| IBIS file was generated by Viper version: 2024.10.21
[IBIS Ver]   4.2
[Comment Char]   |_char
[File Name]   mcxl20_100lqfp_14x14_l25x_tfme.ibs
[File Rev]   1.0
[Date]   Thu Oct 24 12:27:42 2024
[Source]   NXP Viper 2024.10.21
[Notes]
[Disclaimer] IMPORTANT NOTICE
  This information is provided on an AS IS basis and without warranty.
  IN NO EVENT SHALL NXP BE LIABLE FOR INCIDENTAL OR CONSEQUENTIAL
  DAMAGES ARISING FROM USE OF THIS INFORMATION. THIS DISCLAIMER OF
  WARRANTY EXTENDS TO THE USER OF THE INFORMATION, AND TO THEIR CUSTOMERS
  OR USERS OF PRODUCTS  AND IS IN LIEU OF ALL WARRANTIES WHETHER EXPRESS,
  IMPLIED, OR STATUTORY, INCLUDING IMPLIED WARRANTIES OF MERCHANTABILITY
  OR FITNESS FOR PARTICULAR PURPOSE.
  NXP does not represent or warrant that the information furnished
  hereunder is free of infringement of any third party patents,
  copyrights, trade secrets, or other intellectual property rights.
  NXP does not represent or warrant that the information is free of
  defect, or that it meets any particular standard, requirements or need
  of the user of the infomation or their customers.
  NXP reserves the right to change the information in this file
  without notice.
   http://www.nxp.com
[Copyright]   (C) Copyright NXP 2004 - 2024, All Rights Reserved.
|   MCXL20_100LQFP_14x14_L25x_TFME
[Component]   MCXL20_100LQFP_14x14_L25x_TFME
[Manufacturer]   NXP
[Package]
| variable   typ   min   max
R_pkg   0.30564   0.12887   0.35737
L_pkg   5.061e-09   3.022e-09   6.217e-09
C_pkg   1.277e-12   9.885e-13   1.603e-12
[Pin] signal_name   model_name   R_pin   L_pin   C_pin
1   P1_15   a_ip_io_3v_3p3v   0.34361   5.739e-09 1.392e-12
2   P1_16   a_ip_io_3v_3p3v   0.33129   5.397e-09 1.564e-12
3   P1_17   a_ip_io_3v_3p3v   0.33122   5.046e-09 1.446e-12
4   VDD   POWER   NA   NA   NA
5   P1_18   a_ip_io_3v_3p3v   0.33259   4.954e-09 1.335e-12
6   P1_19   a_ip_io_3v_3p3v   0.32237   5.168e-09 1.289e-12
7   P1_20   a_ip_io_3v_3p3v   0.30216   5.026e-09 1.237e-12
8   P1_21   a_ip_io_3v_3p3v   0.29683   4.978e-09 1.206e-12
9   P1_22   a_ip_io_3v_3p3v   0.29435   4.952e-09 1.177e-12
10   P2_0   a_ip_io_3v_3p3v   0.29406   4.947e-09 1.149e-12
11   P2_1   a_ip_io_3v_3p3v   0.29668   4.979e-09 1.095e-12
12   P2_2   a_ip_io_3v_3p3v   0.30138   4.867e-09 1.083e-12
13   P2_3   a_ip_io_3v_3p3v   0.30845   4.904e-09 1.063e-12
14   P2_4   a_ip_io_3v_3p3v   0.30483   4.804e-09 9.885e-13
15   P2_5   a_ip_io_3v_3p3v   0.30153   4.504e-09 1.003e-12
16   VDD   POWER   NA   NA   NA
17   VSS   GND   NA   NA   NA
18   VDD_CORE_FIXED   POWER   NA   NA   NA
19   P2_6   a_ip_io_3v_3p3v   0.31199   4.646e-09 1.139e-12
20   P2_7   a_ip_io_3v_3p3v   0.31342   4.987e-09 1.226e-12
21   P2_10   a_ip_io_3v_3p3v   0.30413   5.068e-09 1.266e-12
22   P2_11   a_ip_io_3v_3p3v   0.31487   5.260e-09 1.245e-12
23   P2_12   a_ip_io_3v_3p3v   0.31693   5.315e-09 1.349e-12
24   P2_13   a_ip_io_3v_3p3v   0.31822   5.354e-09 1.506e-12
25   P2_14   a_ip_io_3v_3p3v   0.33148   5.617e-09 1.387e-12
26   P2_15   a_ip_io_3v_3p3v   0.33786   5.719e-09 1.380e-12
27   P2_16   a_ip_io_3v_3p3v   0.31339   5.264e-09 1.544e-12
28   P2_17   a_ip_io_3v_3p3v   0.3118   5.209e-09 1.436e-12
29   P2_18   a_ip_io_3v_3p3v   0.30788   5.060e-09 1.333e-12
30   P2_19   a_ip_io_3v_3p3v   0.31046   4.771e-09 1.313e-12
31   VDD   POWER   NA   NA   NA
32   VDD_CORE_FIXED   POWER   NA   NA   NA
33   P2_20   NC   0.29722   4.575e-09 1.197e-12
34   P2_21   a_ip_io_3v_3p3v   0.29247   4.706e-09 1.175e-12
35   P2_22   a_ip_io_3v_3p3v   0.29166   4.730e-09 1.148e-12
36   P2_23   a_ip_io_3v_3p3v   0.29368   4.774e-09 1.094e-12
37   P2_24   a_ip_io_3v_3p3v   0.30194   4.871e-09 1.080e-12
38   P2_25   a_ip_io_3v_3p3v   0.3094   4.870e-09 1.049e-12
39   VDD_ANA   POWER   NA   NA   NA
40   VSS   GND   NA   NA   NA
41   VDD   POWER   NA   NA   NA
42   P3_0   NC   0.29643   4.577e-09 1.076e-12
43   P3_1   NC   0.29142   4.749e-09 1.109e-12
44   P3_2   NC   0.30359   4.974e-09 1.132e-12
45   P3_3   NC   0.30687   5.055e-09 1.231e-12
46   P3_4   NC   0.30318   5.083e-09 1.274e-12
47   P3_5   a_ip_io_3v_3p3v   0.31144   5.258e-09 1.248e-12
48   P3_6   a_ip_io_3v_3p3v   0.31786   5.373e-09 1.344e-12
49   P3_9   a_ip_io_3v_3p3v   0.31677   5.604e-09 1.497e-12
50   P3_10   a_ip_io_3v_3p3v   0.34936   6.017e-09 1.380e-12
51   P3_11   a_ip_io_3v_3p3v   0.3307   5.510e-09 1.408e-12
52   P3_12   a_ip_io_3v_3p3v   0.31802   5.253e-09 1.602e-12
53   P3_13   a_ip_io_3v_3p3v   0.3165   5.183e-09 1.488e-12
54   P3_14   a_ip_io_3v_3p3v   0.31608   5.069e-09 1.384e-12
55   P3_15   a_ip_io_3v_3p3v   0.31686   4.693e-09 1.373e-12
56   VDD   POWER   NA   NA   NA
57   VDD_BAT   POWER   NA   NA   NA
58   DCDC_BUCK_LX_FIXED   NC   0.12887   3.022e-09 1.506e-12
59   VSS_DCDC_BUCK   GND   NA   NA   NA
60   DCDC_BUCK_LX_AON   NC   0.1302   3.109e-09 1.407e-12
61   VDD   POWER   NA   NA   NA
62   VSS   GND   NA   NA   NA
63   VDD_CORE_AON   POWER   NA   NA   NA
64   VOUT_RTC   POWER   0.21062   4.052e-09 1.147e-12
65   VOUT_SNS   POWER   0.19819   4.340e-09 1.108e-12
66   P0_0   NC   0.2943   4.858e-09 1.093e-12
67   P0_1   NC   0.29219   5.023e-09 1.130e-12
68   P0_2   NC   0.29215   5.052e-09 1.158e-12
69   P0_3   a_ip_io_3v_3p3v   0.30626   5.232e-09 1.180e-12
70   P0_4   a_ip_io_3v_3p3v   0.31104   5.298e-09 1.279e-12
71   POR_EXT_B   NC   0.31148   5.350e-09 1.321e-12
72   ATESTMODE   NC   0.32593   5.383e-09 1.296e-12
73   RTC_XI   NC   0.3269   5.412e-09 1.397e-12
74   RTC_XO   NC   0.3209   5.507e-09 1.546e-12
75   RESET_B   NC   0.34003   5.961e-09 1.403e-12
76   P0_5   a_ip_io_3v_3p3v   0.35268   6.119e-09 1.411e-12
77   P0_6   a_ip_io_3v_3p3v   0.32741   5.758e-09 1.603e-12
78   P0_7   a_ip_io_3v_3p3v   0.32142   5.634e-09 1.489e-12
79   P0_8   a_ip_io_3v_3p3v   0.31587   5.268e-09 1.386e-12
80   P0_9   a_ip_io_3v_3p3v   0.31043   5.135e-09 1.374e-12
81   P0_10   a_ip_io_3v_3p3v   0.30966   5.073e-09 1.332e-12
82   P0_11   a_ip_io_3v_3p3v   0.2952   4.783e-09 1.282e-12
83   P0_12   a_ip_io_3v_3p3v   0.29955   4.462e-09 1.232e-12
84   VSS   GND   NA   NA   NA
85   VDD_ANA_LPADC   POWER   NA   NA   NA
86   P0_13   a_ip_io_3v_3p3v   0.30364   4.501e-09 1.147e-12
87   P0_14   a_ip_io_3v_3p3v   0.3066   4.775e-09 1.133e-12
88   P0_15   a_ip_io_3v_3p3v   0.31475   4.941e-09 1.115e-12
89   P0_16   a_ip_io_3v_3p3v   0.31436   4.938e-09 1.044e-12
90   P0_17   a_ip_io_3v_3p3v   0.3116   4.656e-09 1.056e-12
91   VDD   POWER   NA   NA   NA
92   P1_0   a_ip_io_3v_3p3v   0.30515   4.688e-09 1.130e-12
93   P1_1   a_ip_io_3v_3p3v   0.30077   4.918e-09 1.158e-12
94   P1_2   a_ip_io_3v_3p3v   0.31333   5.178e-09 1.184e-12
95   P1_3   a_ip_io_3v_3p3v   0.31636   5.252e-09 1.275e-12
96   P1_6   NC   0.30739   5.206e-09 1.315e-12
97   P1_7   NC   0.31882   5.389e-09 1.286e-12
98   P1_10   a_ip_io_3v_3p3v   0.31504   5.361e-09 1.386e-12
99   P1_11   a_ip_io_3v_3p3v   0.32078   5.680e-09 1.544e-12
100   P1_12   NC   0.35737   6.217e-09 1.398e-12
[Pin Mapping]   pulldown_ref   pullup_ref
1   NC   NC
2   NC   NC
3   NC   NC
4   NC   VDD
5   NC   NC
6   NC   NC
7   NC   NC
8   NC   NC
9   NC   NC
10   NC   NC
11   NC   NC
12   NC   NC
13   NC   NC
14   NC   NC
15   NC   NC
16   NC   VDD
17   VSS   NC
18   NC   VDD_CORE_FIXED
19   NC   NC
20   NC   NC
21   NC   NC
22   NC   NC
23   NC   NC
24   NC   NC
25   NC   NC
26   NC   NC
27   NC   NC
28   NC   NC
29   NC   NC
30   NC   NC
31   NC   VDD
32   NC   VDD_CORE_FIXED
33   NC   NC
34   NC   NC
35   NC   NC
36   NC   NC
37   NC   NC
38   NC   NC
39   NC   VDD_ANA
40   VSS   NC
41   NC   VDD
42   NC   NC
43   NC   NC
44   NC   NC
45   NC   NC
46   NC   NC
47   NC   NC
48   NC   NC
49   NC   NC
50   NC   NC
51   NC   NC
52   NC   NC
53   NC   NC
54   NC   NC
55   NC   NC
56   NC   VDD
57   NC   VDD_BAT
58   NC   NC
59   VSS_DCDC_BUCK   NC
60   NC   NC
61   NC   VDD
62   VSS   NC
63   NC   VDD_CORE_AON
64   NC   VOUT_RTC
65   NC   VOUT_SNS
66   NC   NC
67   NC   NC
68   NC   NC
69   NC   NC
70   NC   NC
71   NC   NC
72   NC   NC
73   NC   NC
74   NC   NC
75   NC   NC
76   NC   NC
77   NC   NC
78   NC   NC
79   NC   NC
80   NC   NC
81   NC   NC
82   NC   NC
83   NC   NC
84   VSS   NC
85   NC   VDD_ANA_LPADC
86   NC   NC
87   NC   NC
88   NC   NC
89   NC   NC
90   NC   NC
91   NC   VDD
92   NC   NC
93   NC   NC
94   NC   NC
95   NC   NC
96   NC   NC
97   NC   NC
98   NC   NC
99   NC   NC
100   NC   NC
|*   Model Selector   *
[Model Selector] a_ip_io_3v_3p3v
p_io_25mhz_ds0_sr0_3p3v_mio   dse=0 sre=0 25mhz
p_io_25mhz_ds0_sr1_3p3v_mio   dse=0 sre=1 25mhz
p_io_25mhz_ds1_sr0_3p3v_mio   dse=1 sre=0 25mhz
p_io_25mhz_ds1_sr1_3p3v_mio   dse=1 sre=1 25mhz
p_io_25mhz_r40_ds0_sr0_3p3v_mio   dse=0 sre=0 25mhz_r40
p_io_25mhz_r40_ds0_sr1_3p3v_mio   dse=0 sre=1 25mhz_r40
p_io_25mhz_r40_ds1_sr0_3p3v_mio   dse=1 sre=0 25mhz_r40
p_io_25mhz_r40_ds1_sr1_3p3v_mio   dse=1 sre=1 25mhz_r40
p_io_50mhz_ds0_sr0_3p3v_mio   dse=0 sre=0 50mhz
p_io_50mhz_ds0_sr1_3p3v_mio   dse=0 sre=1 50mhz
p_io_50mhz_ds1_sr0_3p3v_mio   dse=1 sre=0 50mhz
p_io_50mhz_ds1_sr1_3p3v_mio   dse=1 sre=1 50mhz
p_io_25mhz_cap_ds0_sr0_3p3v_mio   dse=0 sre=0 25mhz_cap
p_io_25mhz_cap_ds0_sr1_3p3v_mio   dse=0 sre=1 25mhz_cap
p_io_25mhz_cap_ds1_sr0_3p3v_mio   dse=1 sre=0 25mhz_cap
p_io_25mhz_cap_ds1_sr1_3p3v_mio   dse=1 sre=1 25mhz_cap
p_io_25mhz_2mux_ds0_sr0_3p3v_mio   dse=0 sre=0 25mhz_2mux
p_io_25mhz_2mux_ds0_sr1_3p3v_mio   dse=0 sre=1 25mhz_2mux
p_io_25mhz_2mux_ds1_sr0_3p3v_mio   dse=1 sre=0 25mhz_2mux
p_io_25mhz_2mux_ds1_sr1_3p3v_mio   dse=1 sre=1 25mhz_2mux
p_io_100mhz_ds0_sr0_3p3v_mio   dse=0 sre=0 100mhz
p_io_100mhz_ds0_sr1_3p3v_mio   dse=0 sre=1 100mhz
p_io_100mhz_ds1_sr0_3p3v_mio   dse=1 sre=0 100mhz
p_io_100mhz_ds1_sr1_3p3v_mio   dse=1 sre=1 100mhz
p_io_100mhz_weftd_ds0_sr0_3p3v_mio   dse=0 sre=0 100mhz
p_io_100mhz_weftd_ds0_sr1_3p3v_mio   dse=0 sre=1 100mhz
p_io_100mhz_weftd_ds1_sr0_3p3v_mio   dse=1 sre=0 100mhz
p_io_100mhz_weftd_ds1_sr1_3p3v_mio   dse=1 sre=1 100mhz
p_io_i2c_ds00_ds10_sr0_3p3v_mio   dse0=0 dse1=0 sre=0 i2c
p_io_i2c_ds00_ds10_sr1_3p3v_mio   dse0=0 dse1=0 sre=1 i2c
p_io_i2c_ds00_ds11_sr0_3p3v_mio   dse0=0 dse1=1 sre=0 i2c
p_io_i2c_ds00_ds11_sr1_3p3v_mio   dse0=0 dse1=1 sre=1 i2c
p_io_i2c_ds01_ds10_sr0_3p3v_mio   dse0=1 dse1=0 sre=0 i2c
p_io_i2c_ds01_ds10_sr1_3p3v_mio   dse0=1 dse1=0 sre=1 i2c
p_io_i2c_ds01_ds11_sr0_3p3v_mio   dse0=1 dse1=1 sre=0 i2c
p_io_i2c_ds01_ds11_sr1_3p3v_mio   dse0=1 dse1=1 sre=1 i2c
p_io_i2c_i2c1_3p3v_mio   ipp_i2c_lv=1 i2c
p_io_i2cfmp_ds00_ds10_sr0_3p3v_mio   dse0=0 dse1=0 sre=0 i2cfmp
p_io_i2cfmp_ds00_ds10_sr1_3p3v_mio   dse0=0 dse1=0 sre=1 i2cfmp
p_io_i2cfmp_ds00_ds11_sr0_3p3v_mio   dse0=0 dse1=1 sre=0 i2cfmp
p_io_i2cfmp_ds00_ds11_sr1_3p3v_mio   dse0=0 dse1=1 sre=1 i2cfmp
p_io_i2cfmp_ds01_ds10_sr0_3p3v_mio   dse0=1 dse1=0 sre=0 i2cfmp
p_io_i2cfmp_ds01_ds10_sr1_3p3v_mio   dse0=1 dse1=0 sre=1 i2cfmp
p_io_i2cfmp_ds01_ds11_sr0_3p3v_mio   dse0=1 dse1=1 sre=0 i2cfmp
p_io_i2cfmp_ds01_ds11_sr1_3p3v_mio   dse0=1 dse1=1 sre=1 i2cfmp
p_io_i2cfmp_i2c1_3p3v_mio   ipp_i2c_lv=1 i2cfmp
p_io_rst_3p3v_mio   rst
p_io_rst_rx1p8v_3p3v_mio   rst
p_io_aon_3p3v_mio   rst
| End [Component] MCXL20_100LQFP_14x14_L25x_TFME
| Models and submodels in the file (49): p_io_100mhz_ds0_sr0_3p3v_mio (I/O), p_io_100mhz_ds0_sr1_3p3v_mio (I/O), p_io_100mhz_ds1_sr0_3p3v_mio (I/O), p_io_100mhz_ds1_sr1_3p3v_mio (I/O), p_io_100mhz_weftd_ds0_sr0_3p3v_mio (I/O), p_io_100mhz_weftd_ds0_sr1_3p3v_mio (I/O), p_io_100mhz_weftd_ds1_sr0_3p3v_mio (I/O), p_io_100mhz_weftd_ds1_sr1_3p3v_mio (I/O), p_io_25mhz_2mux_ds0_sr0_3p3v_mio (I/O), p_io_25mhz_2mux_ds0_sr1_3p3v_mio (I/O), p_io_25mhz_2mux_ds1_sr0_3p3v_mio (I/O), p_io_25mhz_2mux_ds1_sr1_3p3v_mio (I/O), p_io_25mhz_cap_ds0_sr0_3p3v_mio (I/O), p_io_25mhz_cap_ds0_sr1_3p3v_mio (I/O), p_io_25mhz_cap_ds1_sr0_3p3v_mio (I/O), p_io_25mhz_cap_ds1_sr1_3p3v_mio (I/O), p_io_25mhz_ds0_sr0_3p3v_mio (I/O), p_io_25mhz_ds0_sr1_3p3v_mio (I/O), p_io_25mhz_ds1_sr0_3p3v_mio (I/O), p_io_25mhz_ds1_sr1_3p3v_mio (I/O), p_io_25mhz_r40_ds0_sr0_3p3v_mio (I/O), p_io_25mhz_r40_ds0_sr1_3p3v_mio (I/O), p_io_25mhz_r40_ds1_sr0_3p3v_mio (I/O), p_io_25mhz_r40_ds1_sr1_3p3v_mio (I/O), p_io_50mhz_ds0_sr0_3p3v_mio (I/O), p_io_50mhz_ds0_sr1_3p3v_mio (I/O), p_io_50mhz_ds1_sr0_3p3v_mio (I/O), p_io_50mhz_ds1_sr1_3p3v_mio (I/O), p_io_aon_3p3v_mio (I/O), p_io_i2c_ds00_ds10_sr0_3p3v_mio (I/O), p_io_i2c_ds00_ds10_sr1_3p3v_mio (I/O), p_io_i2c_ds00_ds11_sr0_3p3v_mio (I/O), p_io_i2c_ds00_ds11_sr1_3p3v_mio (I/O), p_io_i2c_ds01_ds10_sr0_3p3v_mio (I/O), p_io_i2c_ds01_ds10_sr1_3p3v_mio (I/O), p_io_i2c_ds01_ds11_sr0_3p3v_mio (I/O), p_io_i2c_ds01_ds11_sr1_3p3v_mio (I/O), p_io_i2c_i2c1_3p3v_mio (I/O), p_io_i2cfmp_ds00_ds10_sr0_3p3v_mio (I/O), p_io_i2cfmp_ds00_ds10_sr1_3p3v_mio (I/O), p_io_i2cfmp_ds00_ds11_sr0_3p3v_mio (I/O), p_io_i2cfmp_ds00_ds11_sr1_3p3v_mio (I/O), p_io_i2cfmp_ds01_ds10_sr0_3p3v_mio (I/O), p_io_i2cfmp_ds01_ds10_sr1_3p3v_mio (I/O), p_io_i2cfmp_ds01_ds11_sr0_3p3v_mio (I/O), p_io_i2cfmp_ds01_ds11_sr1_3p3v_mio (I/O), p_io_i2cfmp_i2c1_3p3v_mio (I/O), p_io_rst_3p3v_mio (I/O), p_io_rst_rx1p8v_3p3v_mio (I/O)
